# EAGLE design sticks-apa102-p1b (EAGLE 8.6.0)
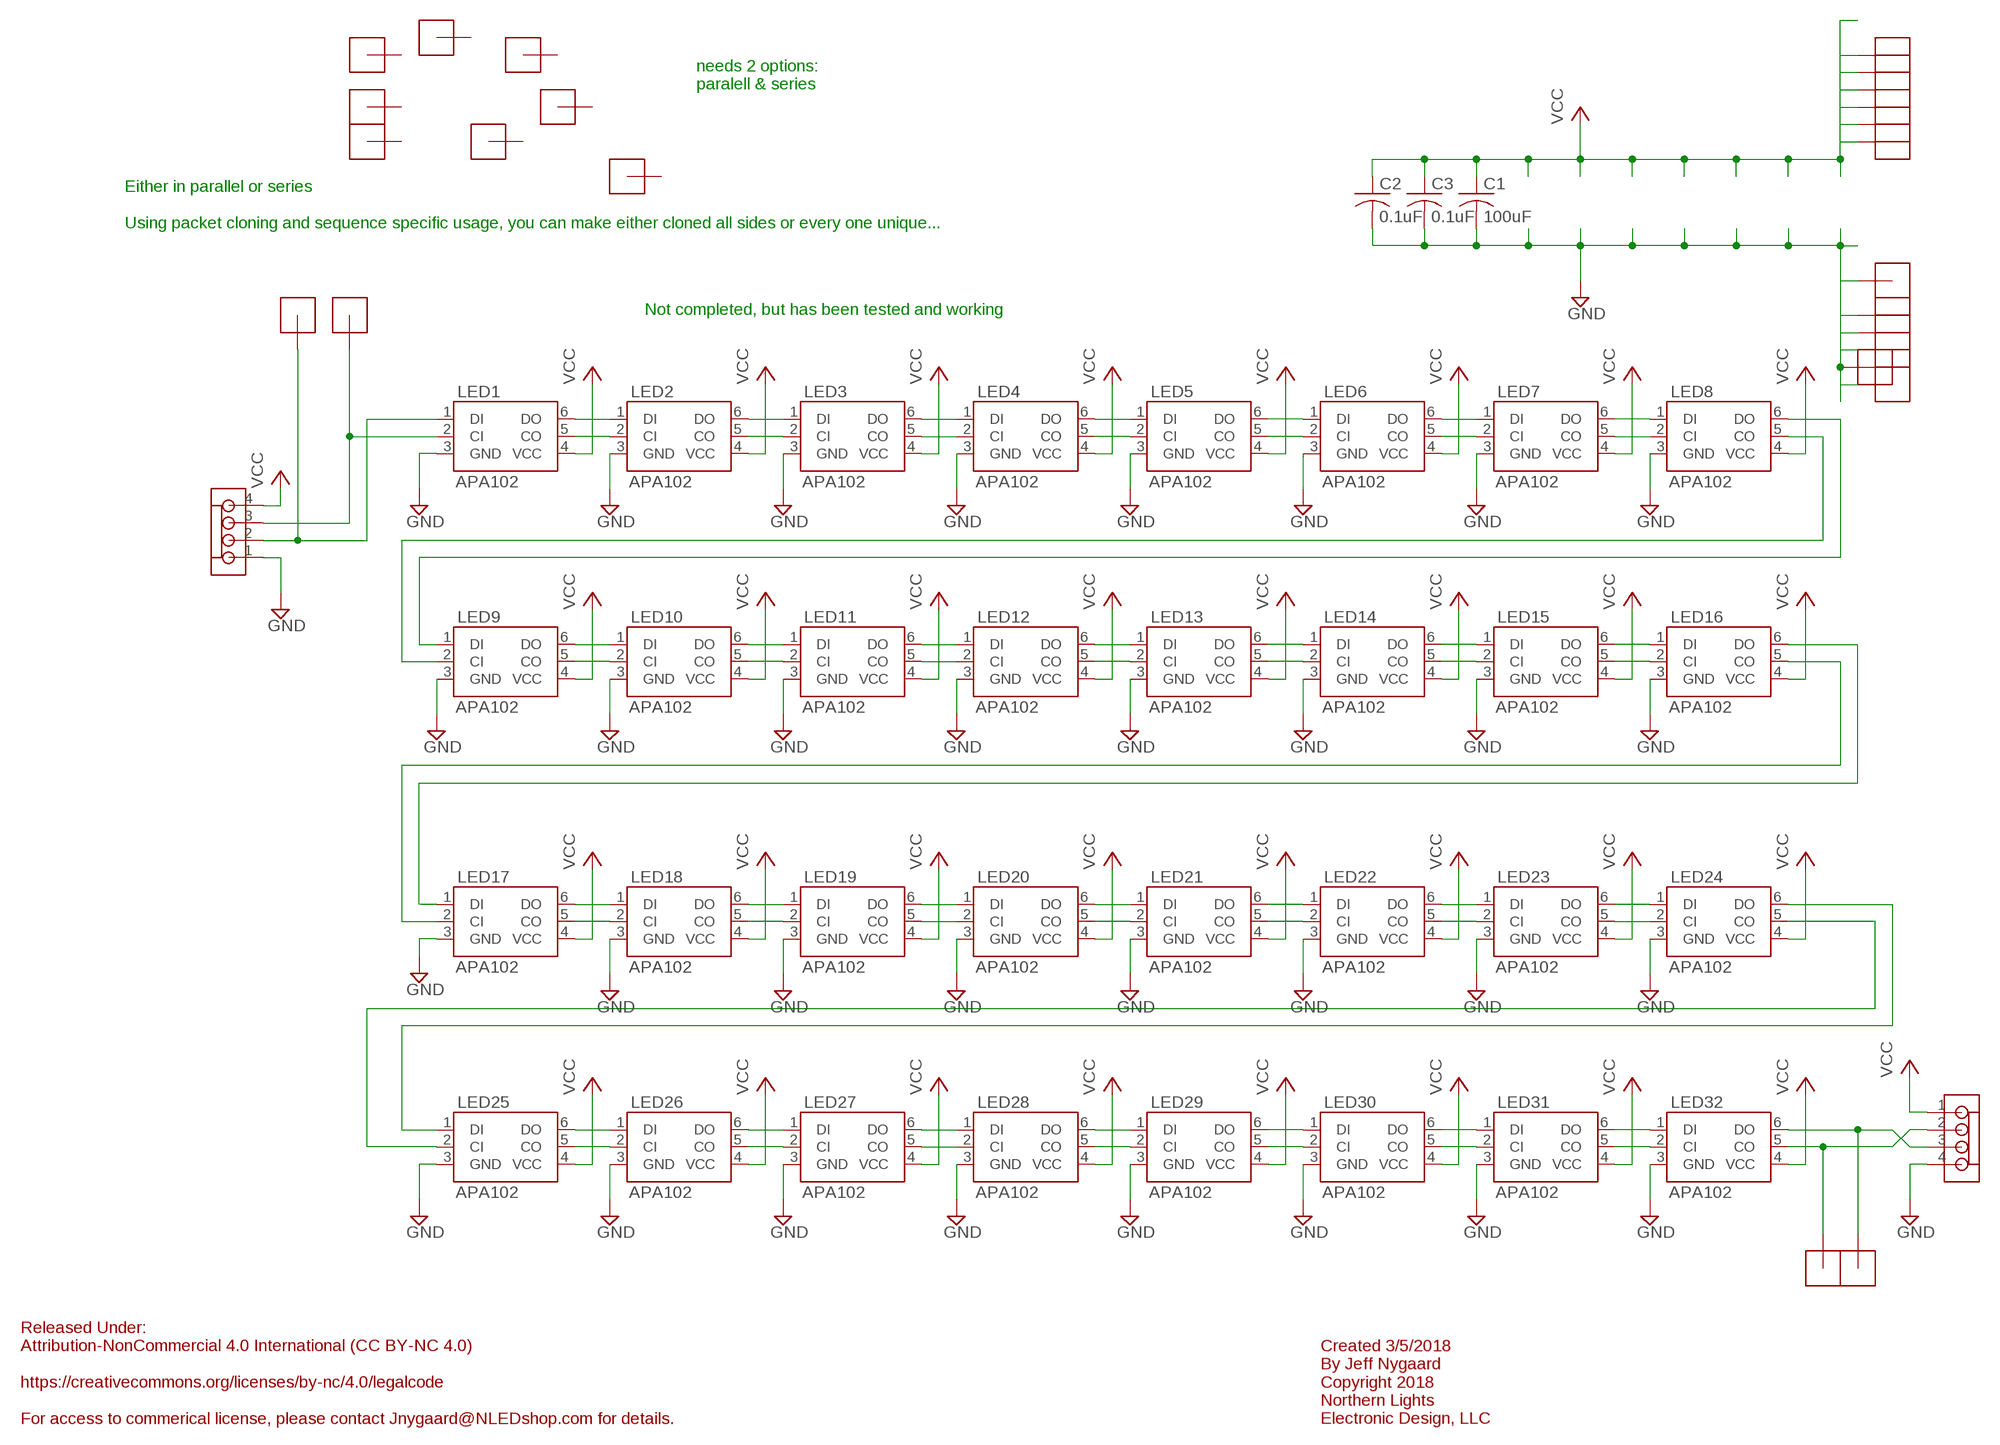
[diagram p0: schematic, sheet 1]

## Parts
C1  100uF  C-USC1206  [C1206]
C2  0.1uF  C-USC1206  [C1206]
C3  0.1uF  C-USC1206  [C1206]
CLKI  1HEADER  [J1]
CLKO  1HEADER  [J1]
DATI  1HEADER  [J1]
DATO  1HEADER  [J1]
IN  MOLEXKK4  [MOLEXKK4]
JGND1  1HEADER  [J1]
JGND2  1HEADER  [J1]
JGND3  1HEADER  [J1]
JGND4  1HEADER  [J1]
JGND5  1HEADER  [J1]
JGND6  1HEADER  [J1]
JVCC1  1HEADER  [J1]
JVCC2  1HEADER  [J1]
JVCC3  1HEADER  [J1]
JVCC4  1HEADER  [J1]
JVCC5  1HEADER  [J1]
JVCC6  1HEADER  [J1]
LED1  APA102  [APA102]
LED2  APA102  [APA102]
LED3  APA102  [APA102]
LED4  APA102  [APA102]
LED5  APA102  [APA102]
LED6  APA102  [APA102]
LED7  APA102  [APA102]
LED8  APA102  [APA102]
LED9  APA102  [APA102]
LED10  APA102  [APA102]
LED11  APA102  [APA102]
LED12  APA102  [APA102]
LED13  APA102  [APA102]
LED14  APA102  [APA102]
LED15  APA102  [APA102]
LED16  APA102  [APA102]
LED17  APA102  [APA102]
LED18  APA102  [APA102]
LED19  APA102  [APA102]
LED20  APA102  [APA102]
LED21  APA102  [APA102]
LED22  APA102  [APA102]
LED23  APA102  [APA102]
LED24  APA102  [APA102]
LED25  APA102  [APA102]
LED26  APA102  [APA102]
LED27  APA102  [APA102]
LED28  APA102  [APA102]
LED29  APA102  [APA102]
LED30  APA102  [APA102]
LED31  APA102  [APA102]
LED32  APA102  [APA102]
M1  1HEADER  [J1]
M2  1HEADER  [J1]
M3  1HEADER  [J1]
M4  1HEADER  [J1]
M5  1HEADER  [J1]
M6  1HEADER  [J1]
M7  1HEADER  [J1]
M8  1HEADER  [J1]
OUT  MOLEXKK4  [MOLEXKK4]

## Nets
GND: C1.2 C2.2 C3.2 IN.1 JGND1.2(J1) JGND2.2(J1) JGND3.2(J1) JGND4.2(J1) JGND5.2(J1) JGND6.2(J1) LED1.3(GND) LED2.3(GND) LED3.3(GND) LED4.3(GND) LED5.3(GND) LED6.3(GND) LED7.3(GND) LED8.3(GND) LED9.3(GND) LED10.3(GND) LED11.3(GND) LED12.3(GND) LED13.3(GND) LED14.3(GND) LED15.3(GND) LED16.3(GND) LED17.3(GND) LED18.3(GND) LED19.3(GND) LED20.3(GND) LED21.3(GND) LED22.3(GND) LED23.3(GND) LED24.3(GND) LED25.3(GND) LED26.3(GND) LED27.3(GND) LED28.3(GND) LED29.3(GND) LED30.3(GND) LED31.3(GND) LED32.3(GND) OUT.4
N$1: LED1.6(DO) LED2.1(DI)
N$2: LED2.6(DO) LED3.1(DI)
N$3: LED3.6(DO) LED4.1(DI)
N$4: LED3.5(CO) LED4.2(CI)
N$5: LED2.5(CO) LED3.2(CI)
N$6: LED1.5(CO) LED2.2(CI)
N$7: LED4.6(DO) LED5.1(DI)
N$8: LED4.5(CO) LED5.2(CI)
N$9: LED5.6(DO) LED6.1(DI)
N$10: LED5.5(CO) LED6.2(CI)
N$11: LED8.5(CO) LED9.2(CI)
N$12: LED8.6(DO) LED9.1(DI)
N$13: LED7.6(DO) LED8.1(DI)
N$14: LED7.5(CO) LED8.2(CI)
N$15: LED6.5(CO) LED7.2(CI)
N$16: LED6.6(DO) LED7.1(DI)
N$17: LED17.6(DO) LED18.1(DI)
N$18: LED18.6(DO) LED19.1(DI)
N$19: LED19.6(DO) LED20.1(DI)
N$20: LED19.5(CO) LED20.2(CI)
N$21: LED18.5(CO) LED19.2(CI)
N$22: LED9.6(DO) LED10.1(DI)
N$23: LED10.6(DO) LED11.1(DI)
N$24: LED11.6(DO) LED12.1(DI)
N$25: LED11.5(CO) LED12.2(CI)
N$26: LED10.5(CO) LED11.2(CI)
N$27: LED9.5(CO) LED10.2(CI)
N$28: LED12.6(DO) LED13.1(DI)
N$29: LED12.5(CO) LED13.2(CI)
N$30: LED13.6(DO) LED14.1(DI)
N$31: LED13.5(CO) LED14.2(CI)
N$32: LED14.6(DO) LED15.1(DI)
N$33: LED14.5(CO) LED15.2(CI)
N$34: LED15.6(DO) LED16.1(DI)
N$35: LED15.5(CO) LED16.2(CI)
N$36: LED17.5(CO) LED18.2(CI)
N$37: LED20.6(DO) LED21.1(DI)
N$38: LED20.5(CO) LED21.2(CI)
N$39: LED21.6(DO) LED22.1(DI)
N$40: LED21.5(CO) LED22.2(CI)
N$41: LED25.6(DO) LED26.1(DI)
N$42: LED26.6(DO) LED27.1(DI)
N$43: LED27.6(DO) LED28.1(DI)
N$44: LED27.5(CO) LED28.2(CI)
N$45: LED26.5(CO) LED27.2(CI)
N$46: LED25.5(CO) LED26.2(CI)
N$47: LED28.6(DO) LED29.1(DI)
N$48: LED28.5(CO) LED29.2(CI)
N$49: LED29.6(DO) LED30.1(DI)
N$50: LED29.5(CO) LED30.2(CI)
N$51: LED30.6(DO) LED31.1(DI)
N$52: LED30.5(CO) LED31.2(CI)
N$53: LED31.6(DO) LED32.1(DI)
N$54: LED31.5(CO) LED32.2(CI)
N$55: LED23.6(DO) LED24.1(DI)
N$56: LED23.5(CO) LED24.2(CI)
N$57: LED22.5(CO) LED23.2(CI)
N$58: LED22.6(DO) LED23.1(DI)
N$59: LED24.6(DO) LED25.1(DI)
N$60: LED24.5(CO) LED25.2(CI)
N$61: LED16.5(CO) LED17.2(CI)
N$62: DATO.2(J1) LED32.6(DO) OUT.3
N$63: CLKO.2(J1) LED32.5(CO) OUT.2
N$87: LED16.6(DO) LED17.1(DI)
N$122: DATI.2(J1) IN.2 LED1.1(DI)
N$123: CLKI.2(J1) IN.3 LED1.2(CI)
VCC: C1.1 C2.1 C3.1 IN.4 JVCC1.2(J1) JVCC2.2(J1) JVCC3.2(J1) JVCC4.2(J1) JVCC5.2(J1) JVCC6.2(J1) LED1.4(VCC) LED2.4(VCC) LED3.4(VCC) LED4.4(VCC) LED5.4(VCC) LED6.4(VCC) LED7.4(VCC) LED8.4(VCC) LED9.4(VCC) LED10.4(VCC) LED11.4(VCC) LED12.4(VCC) LED13.4(VCC) LED14.4(VCC) LED15.4(VCC) LED16.4(VCC) LED17.4(VCC) LED18.4(VCC) LED19.4(VCC) LED20.4(VCC) LED21.4(VCC) LED22.4(VCC) LED23.4(VCC) LED24.4(VCC) LED25.4(VCC) LED26.4(VCC) LED27.4(VCC) LED28.4(VCC) LED29.4(VCC) LED30.4(VCC) LED31.4(VCC) LED32.4(VCC) OUT.1
Unconnected: M1.2(J1) M2.2(J1) M3.2(J1) M4.2(J1) M5.2(J1) M6.2(J1) M7.2(J1) M8.2(J1)

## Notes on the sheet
- needs 2 options:
  paralell & series
- Either in parallel or series
  
  Using packet cloning and sequence specific usage, you can make either cloned all sides or every one unique...
- Not completed, but has been tested and working
- Released Under:
  Attribution-NonCommercial 4.0 International (CC BY-NC 4.0)
  
  https://creativecommons.org/licenses/by-nc/4.0/legalcode
  
  For access to commerical license, please contact Jnygaard@NLEDshop.com for details.
- Created 3/5/2018
  By Jeff Nygaard
  Copyright 2018
  Northern Lights
  Electronic Design, LLC

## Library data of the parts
C1-C3 = rcl:C-US: CAPACITOR, American symbol
CLKI CLKO DATI DATO JGND1-JGND6 JVCC1-JVCC6 M1-M8 = ChromationSystems-1:1HEADER
IN OUT = ChromationSystems-1:MOLEXKK4
LED1-LED32 = ChromationSystems-2:APA102

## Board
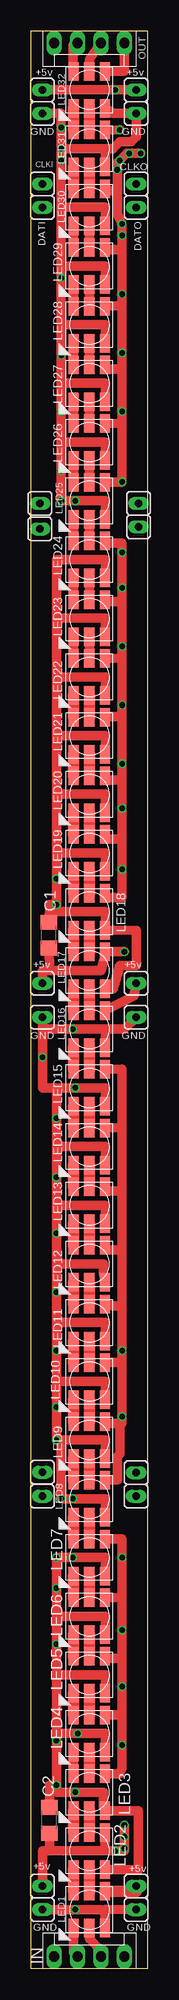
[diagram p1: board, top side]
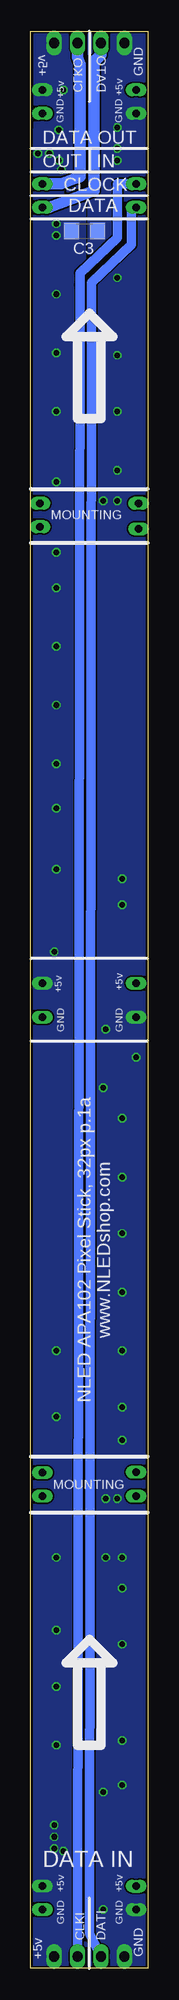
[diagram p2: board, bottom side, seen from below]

Size 12.7 x 209.55 mm. Coordinates in mm from the lower left corner, seen from the top.
Outline: 0,0 12.7,0 12.7,209.55 0,209.55 0,0
Copper layers (1*16): Top 0.035mm / dielectric 1.5mm / Bottom 0.035mm
Design rules "SeeedStudio_2layer_DRU_no_angle_20140221 *": minimum track width 6mil, minimum drill 12mil, track to track 6mil, track to pad 6mil, pad to pad 6mil, via to via 6mil, smd to smd 0mil, copper to edge 10mil, drill to drill 10mil, minimum pad ring 10mil, minimum via ring 6mil, stop-mask expansion 2mil, vias tented up to drill 100mil, thermal gap 10mil

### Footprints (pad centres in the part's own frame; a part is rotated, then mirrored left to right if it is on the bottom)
C1206 = smd 1.6 x 1.8: 1 -1.4,0; 2 1.4,0
J1 = drill 0.813 pad 1.422 long: 2 0,0
MOLEXKK4 = drill 1.1 long: 1 -3.81,0; 2 -1.27,0; 3 1.27,0; 4 3.81,0
APA102 = smd 2 x 1.1: 1 -2,1.7; 2 -2,0; 3 -2,-1.7; 4 2,-1.7; 5 2,0; 6 2,1.7

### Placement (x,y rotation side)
C1  1.97,111.76 90 top
C2  2.03,16 90 top
C3  6.86,187.96 0 bottom
CLKI  1.27,193.04 0 top
CLKO  11.43,193.04 0 top
DATI  1.27,190.5 0 top
DATO  11.43,190.5 0 top
IN  6.35,1.27 0 top
JGND1  1.27,6.35 180 top
JGND2  11.43,6.35 0 top
JGND3  1.27,200.66 0 top
JGND4  11.43,200.66 0 top
JGND5  1.27,102.87 0 top
JGND6  11.43,102.87 0 top
JVCC1  1.27,8.89 180 top
JVCC2  11.43,8.89 0 top
JVCC3  1.27,203.2 0 top
JVCC4  11.43,203.2 0 top
JVCC5  1.27,106.55 0 top
JVCC6  11.43,106.55 0 top
LED1  6.35,6.35 90 top
LED2  6.35,12.7 90 top
LED3  6.35,19.05 90 top
LED4  6.35,25.4 90 top
LED5  6.35,31.75 90 top
LED6  6.35,38.1 90 top
LED7  6.35,44.45 90 top
LED8  6.35,50.8 90 top
LED9  6.35,57.15 90 top
LED10  6.35,63.5 90 top
LED11  6.35,69.85 90 top
LED12  6.35,76.2 90 top
LED13  6.35,82.55 90 top
LED14  6.35,88.9 90 top
LED15  6.35,95.25 90 top
LED16  6.35,101.6 90 top
LED17  6.35,107.95 90 top
LED18  6.35,114.3 90 top
LED19  6.35,120.65 90 top
LED20  6.35,127 90 top
LED21  6.35,133.35 90 top
LED22  6.35,139.7 90 top
LED23  6.35,146.05 90 top
LED24  6.35,152.4 90 top
LED25  6.35,158.75 90 top
LED26  6.35,165.1 90 top
LED27  6.35,171.45 90 top
LED28  6.35,177.8 90 top
LED29  6.35,184.15 90 top
LED30  6.35,190.5 90 top
LED31  6.35,196.85 90 top
LED32  6.35,203.2 90 top
M1  1.27,53.66 0 top
M2  1.27,51.05 0 top
M3  11.43,51.05 0 top
M4  11.43,53.59 0 top
M5  1.02,158.5 0 top
M6  1.02,155.7 0 top
M7  11.68,155.96 0 top
M8  11.68,158.5 0 top
OUT  6.35,208.28 180 top

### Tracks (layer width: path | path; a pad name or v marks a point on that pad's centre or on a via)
GND  (via drill 0.6)
  Top 1.016: JGND2.2 8.16,6.38 LED1.3 8.05,5.92 7.62,6.35 v4.83,6.35 JGND1.2 | 2.79,76.2 7.87,76.2 7.87,75.18 LED12.3 | LED13.3 8.13,81.03 8.13,82.55 2.79,82.55 | 2.79,82.55 v2.79,79.5 2.79,76.2 | LED14.3 8.13,87.38 8.13,88.9 2.79,88.9 | 2.79,88.9 v2.79,85.6 2.79,82.55 | LED15.3 8.13,93.73 8.13,95.25 v4.83,95.25 2.79,95.25 | 2.79,95.25 v2.79,91.95 2.79,88.9 | LED16.3 8.13,101.6 | LED17.3 8.89,105.92 9.65,108.46 11.43,108.46 11.43,112.27 LED18.3 8.13,112.78 8.13,114.3 2.79,114.3 v2.79,115.06 | LED19.3 8.13,119.13 8.13,120.65 2.79,120.65 | 2.79,120.65 v2.79,117.86 v2.79,115.06 | LED20.3 8.13,125.48 8.13,127 2.79,127 | 2.79,127 2.79,120.65 | 2.79,95.25 1.27,95.25 v1.27,98.55 1.27,101.6 | 1.27,101.6 JGND5.2 | 8.13,101.6 v4.57,101.6 1.27,101.6 | 8.13,101.6 10.16,101.6 JGND6.2 | LED2.3 8.13,10.67 11.68,10.67 11.68,17.02 8.13,17.02 LED3.3 7.87,17.53 7.87,19.05 v4.83,19.05 2.79,19.05 v2.79,19.81 | v2.79,19.81 v2.79,24.64 | v2.79,24.64 2.79,25.4 v5.08,25.4 8.13,25.4 LED4.3 | LED6.3 8.13,36.58 8.13,38.1 2.79,38.1 | 2.79,38.1 v2.79,35.05 2.79,31.75 | 2.79,31.75 v2.79,24.64 | LED5.3 8.13,30.23 8.13,31.75 2.79,31.75 | LED7.3 8.13,42.93 8.13,44.45 v4.57,44.45 v2.79,44.45 v2.79,41.15 2.79,38.1 | LED8.3 8.13,49.28 8.13,50.8 v4.57,50.8 v3.3,50.8 3.3,57.15 | LED9.3 8.13,55.63 8.13,57.15 3.3,57.15 | 3.3,57.15 v2.79,57.15 v2.79,60.71 2.79,63.5 | LED10.3 8.13,61.98 8.13,63.5 2.79,63.5 | 2.79,76.2 v2.79,73.15 2.79,69.85 | 2.79,69.85 v2.79,66.8 2.79,63.5 | LED11.3 8.13,68.33 8.13,69.85 2.79,69.85 | LED21.3 8.13,131.57 8.13,133.35 2.79,133.35 | 2.79,127 2.79,133.35 | 2.79,133.35 2.79,139.7 | 2.79,139.7 2.79,146.05 | 2.79,146.05 2.79,152.4 8.13,152.4 8.13,150.62 LED24.3
  Top 1.016: LED22.3 8.13,138.18 8.13,139.7 2.79,139.7 | LED23.3 8.13,144.53 8.13,146.05 2.79,146.05 | LED25.3 8.13,157.23 8.13,158.75 v4.83,158.75 v3.3,158.75 v3.3,162.05 3.3,165.1 | LED26.3 8.13,163.58 8.13,165.1 3.3,165.1 | LED27.3 8.13,169.93 8.13,171.45 3.3,171.45 | LED31.3 8.13,195.07 8.13,196.85 | v3.3,196.85 v3.3,195.58 3.3,190.5 | 3.3,190.5 3.3,184.15 | 3.3,184.15 v3.3,182.88 3.3,177.8 | 3.3,177.8 v3.3,174.5 3.3,171.45 | 3.3,171.45 v3.3,168.4 3.3,165.1 | LED29.3 8.13,182.37 8.13,184.15 3.3,184.15 | v3.3,196.85 8.13,196.85 | LED28.3 8.13,176.28 8.13,177.8 3.3,177.8 | LED30.3 8.13,188.98 8.13,190.5 3.3,190.5 | LED32.3 8.89,200.66 JGND4.2 11.43,198.12 10.92,197.61 9.65,197.61 8.89,196.85 8.13,196.85 | v3.3,196.85 v3.3,199.14 3.3,200.66 JGND3.2 | C1.2 2.03,115.06 v2.79,115.06 | C2.2 2.03,19.81 v2.79,19.81
  pour Bottom (no thermals): 0,209.55 0,0 6.35,0 6.35,209.55
N$1
  Top 1.27: LED2.1 LED1.6
N$2
  Top 1.27: LED2.6 LED3.1
N$3
  Top 1.016: LED4.1 LED3.6
N$4
  Top 1.27: LED4.2 LED3.5
N$5
  Top 1.27: LED2.5 LED3.2
N$6
  Top 1.27: LED1.5 LED2.2
N$7
  Top 1.27: LED5.1 LED4.6
N$8
  Top 1.27: LED5.2 LED4.5
N$9
  Top 1.27: LED6.1 LED5.6
N$10
  Top 1.27: LED5.5 LED6.2
N$11
  Top 1.27: LED9.2 LED8.5
N$12
  Top 1.27: LED9.1 LED8.6
N$13
  Top 1.27: LED8.1 LED7.6
N$14
  Top 1.27: LED8.2 LED7.5
N$15
  Top 1.27: LED6.5 LED7.2
N$16
  Top 1.27: LED7.1 LED6.6
N$17
  Top 1.27: LED18.1 LED17.6
N$18
  Top 1.27: LED19.1 LED18.6
N$19
  Top 1.27: LED20.1 LED19.6
N$20
  Top 1.27: LED20.2 LED19.5
N$21
  Top 1.27: LED18.5 LED19.2
N$22
  Top 1.27: LED9.6 LED10.1
N$23
  Top 1.27: LED11.1 LED10.6
N$24
  Top 1.27: LED12.1 LED11.6
N$25
  Top 1.27: LED12.2 LED11.5
N$26
  Top 1.27: LED11.2 LED10.5
N$27
  Top 1.27: LED9.5 LED10.2
N$28
  Top 1.27: LED13.1 LED12.6
N$29
  Top 1.27: LED13.2 LED12.5
N$30
  Top 1.27: LED14.1 LED13.6
N$31
  Top 1.27: LED14.2 LED13.5
N$32
  Top 1.27: LED14.6 LED15.1
N$33
  Top 1.27: LED15.2 LED14.5
N$34
  Top 1.27: LED16.1 LED15.6
N$35
  Top 1.27: LED16.2 LED15.5
N$36
  Top 1.27: LED18.2 LED17.5
N$37
  Top 1.27: LED21.1 LED20.6
N$38
  Top 1.27: LED21.2 LED20.5
N$39
  Top 1.27: LED22.1 LED21.6
N$40
  Top 1.27: LED22.2 LED21.5
N$41
  Top 1.016: LED25.6 LED26.1
N$42
  Top 1.016: LED26.6 LED27.1
N$43
  Top 1.016: LED28.1 LED27.6
N$44
  Top 1.016: LED27.5 LED28.2
N$45
  Top 1.016: LED26.5 LED27.2
N$46
  Top 1.016: LED26.2 LED25.5
N$47
  Top 1.016: LED29.1 LED28.6
N$48
  Top 1.016: LED29.2 LED28.5
N$49
  Top 1.016: LED29.6 LED30.1
N$50
  Top 1.016: LED30.2 LED29.5
N$51
  Top 1.27: LED31.1 LED30.6
N$52
  Top 1.27: LED30.5 LED31.2
N$53
  Top 1.27: LED32.1 LED31.6
N$54
  Top 1.27: LED32.2 LED31.5
N$55
  Top 1.016: LED24.1 LED23.6
N$56
  Top 1.016: LED24.2 LED23.5
N$57
  Top 1.016: LED23.2 LED22.5
N$58
  Top 1.016: LED23.1 LED22.6
N$59
  Top 1.016: LED25.1 LED24.6
N$60
  Top 1.016: LED25.2 LED24.5
N$61
  Top 1.27: LED17.2 LED16.5
N$62
  Top 1.016: LED32.6 4.57,205.74 4.57,208.03 OUT.3
  Bottom 1.27: OUT.3 5.08,207.01 5.84,206.25 5.84,192.28 10.67,190.5 DATO.2
N$63
  Top 1.016: LED32.5 6.35,206.5 OUT.2
  Bottom 1.27: OUT.2 7.62,206.76 7.37,205.99 7.37,193.8 9.4,193.04 CLKO.2
N$87
  Top 1.27: LED17.1 LED16.6
N$122
  Top 1.016: LED1.1 4.65,1.7 IN.2
  Bottom 1.016: DATI.2 1.78,190.5 1.78,186.44 6.1,182.37 6.1,180.85 6.35,3.81 IN.2
N$123
  Top 1.016: LED1.2 6.35,3.17 7.62,1.91 IN.3
  Bottom 1.016: CLKI.2 3.3,193.04 3.3,187.2 7.37,183.39 7.37,182.12 7.62,3.81 IN.3
VCC  (via drill 0.6)
  Top 0.406: v9.91,59.69 9.65,58.42
  Top 1.016: 8.26,8.14 LED1.4 | JVCC1.2 1.27,12.7 2.03,12.7 | 2.03,12.7 8.26,12.7 | 8.26,12.7 v9.14,12.7 10.16,12.7 v10.16,15.49 | LED2.4 8.05,12.9 8.26,12.7 | LED3.4 9.62,21.05 9.91,21.59 v9.91,24.13 9.91,27.18 | LED4.4 8.08,27.43 9.65,27.43 9.91,27.18 | LED5.4 8.16,33.75 8.13,33.53 9.91,33.53 | 9.91,33.53 v9.91,36.58 9.91,40.13 | 9.91,33.53 v9.91,30.48 9.91,27.18 | LED6.4 9.91,40.13 | LED7.4 9.91,46.48 v9.91,44.45 9.91,40.13 | 8.13,58.93 LED9.4 8.13,58.67 8.13,58.93 | 8.13,71.63 LED11.4 8.89,71.63 9.91,71.63 | LED10.4 8.13,65.53 9.91,65.53 | 9.91,65.53 9.91,71.63 | LED12.4 8.38,77.72 9.91,77.72 | 9.91,77.72 9.91,71.63 | LED13.4 8.13,84.07 9.91,84.07 | 9.91,84.07 9.91,77.72 | LED14.4 9.91,90.93 | 9.91,90.93 9.91,84.07 | LED15.4 9.91,97.28 9.91,90.93 | LED17.4 8.13,109.73 | LED18.4 8.13,115.82 9.91,115.82 v9.91,118.87 9.91,122.17 | LED19.4 8.13,122.17 9.91,122.17 | LED20.4 8.13,128.52 9.91,128.52 | 9.91,128.52 v9.91,125.48 9.91,122.17 | 9.91,65.53 v9.91,59.69 9.91,58.93 9.65,58.93 | LED8.4 8.13,52.83 9.4,52.83 9.4,55.37 9.65,55.63 9.65,58.42 9.65,58.93 | 8.13,58.93 9.65,58.93 | 8.13,103.38 8.13,103.12 LED16.4 11.18,105.16 JVCC6.2 | 8.13,109.73 8.13,109.98 v10.16,109.98 | JVCC5.2 1.27,107.95 2.03,107.95 | 2.03,107.95 7.62,107.95 8.13,109.73 | LED21.4 8.13,135.38 9.91,135.38 | 9.91,135.38 9.91,128.52 | LED22.4 9.91,141.73 | 9.91,141.73 9.91,135.38 | LED23.4 8.13,147.83 9.91,147.83 | 9.91,147.83 9.91,141.73 | LED24.4 8.13,154.18 9.91,154.18 9.91,147.83 | LED27.4 8.13,172.97 9.91,172.97 | 9.91,172.97 9.91,167.13 | 9.91,167.13 v9.91,160.78 LED25.4 | LED26.4 9.91,167.13 | LED28.4 9.91,179.83 | 9.91,179.83 9.91,172.97 | LED29.4 8.13,185.93 9.91,185.93
  Top 1.016: 9.91,185.93 9.91,179.83 | 9.91,185.93 v9.91,188.72 9.4,189.74 9.4,192.28 | JVCC3.2 v9.14,203.2 JVCC4.2 | LED31.4 v9.65,198.88 | LED32.4 10.16,205.23 OUT.1 | 9.4,192.28 9.4,195.33 v9.65,195.58 10.41,196.34 v11.94,196.34 | LED30.4 8.13,192.28 9.4,192.28 | C1.1 2.03,107.95 | C2.1 2.03,12.7
  Top 1.27: LED1.4 11.43,8.35 JVCC2.2
  other vias: 9.91,66.8 9.91,136.65 9.91,130.3 9.91,143 9.91,149.35 9.91,153.16 9.91,168.4 9.91,174.75 9.91,181.1 9.91,187.45 10.16,14.22 10.16,12.95 10.67,196.34 9.4,194.56
  pour Bottom (rank 2, no thermals): 6.35,209.55 6.35,0 10.67,-0.25 12.7,-0.25 12.19,209.55

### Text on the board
tNames: +5v | +5v | GND | GND | CLKI | CLKO | DATI | DATO | +5v | +5v | GND | GND | +5v | +5v | GND | GND
bNames: GND | +5v | +5v | +5v | DATO | CLKO | GND | GND | DATA OUT | OUT IN | CLOCK | DATA | MOUNTING | +5v | +5v | GND | GND | NLED APA102 Pixel Stick, 32px p.1a / www.NLEDshop.com | MOUNTING | DATA IN | +5v | +5v | GND | GND | DATI | CLKI | GND | +5v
